| IBIS file stm32l4r5_s5_r7_s7_ufbga169.ibs
[IBIS ver]   4.2
[File name]   stm32l4r5_s5_r7_s7_ufbga169.ibs
[File Rev]   1.0
[Date]   01-6-2017
[Source]   Data Created at STMicroelectronics
[Notes]   File originated from ELDO simulations.
[Disclaimer]  This information is for modeling purpose only and is
   not guaranted.
   The information is subject to change without notice.
[Copyright]   Copyright 2017 STMicroelectronics Inc.
|   Component stm32l4r5_s5_r7_s7_ufbga169
[Component] stm32l4r5_s5_r7_s7_ufbga169
[Manufacturer] STMicroelectronics
[Package]
| variable   typ   min   max
R_pkg   0.0   0.0   0.0
L_pkg   0.0H   0.0H   0.0H
C_pkg   0.0F   0.0F   0.0F
[Pin]  signal_name   model_name   R_pin   L_pin   C_pin
A1 PI10 io8prog2m25m50m120m_sudq_ft
A10 PA14 io8prog2m25m50m120m_sudq_ft
A11 PA13 io8prog2m25m50m120m_sudq_ft
A12 PI0 io8prog2m25m50m120m_sudq_ft
A13 PH14 io8prog2m25m50m120m_sudq_ft
A2 PH2 io8prog2m25m50m120m_sudq_ft
A3 VDD power
A4 PE0 io8prog2m25m50m120m_sudq_ft
A5 PB4 io8prog2m25m50m120m_sudq_i2c_ft
A6 PB3 io8prog2m25m50m120m_sudq_ft
A7 VSS gnd
A8 VDD power
A9 PA15 io8prog2m25m50m120m_sudq_ft
B1 PI9 io8prog2m25m50m120m_sudq_ft
B10 PI2 io8prog2m25m50m120m_sudq_ft
B11 PI1 io8prog2m25m50m120m_sudq_ft
B12 PH15 io8prog2m25m50m120m_sudq_ft
B13 PH12 io8prog2m25m50m120m_sudq_ft
B2 PI7 io8prog2m25m50m120m_sudq_ft
B3 VSS gnd
B4 PE1 io8prog2m25m50m120m_sudq_ft
B5 PB5 io8prog2m25m50m120m_sudq_ft
B6 VDDIO2 power
B7 PG9 io8prog2m25m50m120m_sudq_ft
B8 PD0 io8prog2m25m50m120m_sudq_ft
B9 PI6 io8prog2m25m50m120m_sudq_ft
C1 VDD power
C10 PI3 io8prog2m25m50m120m_sudq_ft
C11 PI8 io8prog2m25m50m120m_sudq_ft
C12 VSS gnd
C13 VDD power
C2 VSS gnd
C3 PI11 io8prog2m25m50m120m_sudq_ft
C4 PB8 io8prog2m25m50m120m_sudq_i2c_ft
C5 PB6 io8prog2m25m50m120m_sudq_i2c_ft
C6 PG15 io8prog2m25m50m120m_sudq_ft
C7 PD4 io8prog2m25m50m120m_sudq_ft
C8 PD1 io8prog2m25m50m120m_sudq_ft
C9 PH13 io8prog2m25m50m120m_sudq_ft
D1 PE4 io8prog2m25m50m120m_sudq_ft
D10 PI4 io8prog2m25m50m120m_sudq_ft
D11 PH9 io8prog2m25m50m120m_sudq_ft
D12 PH7 io8prog2m25m50m120m_sudq_i2c_ft
D13 PA12 io8usblsfs_otg2
D2 PE3 io8prog2m25m50m120m_sudq_ft
D3 PE2 io8prog2m25m50m120m_sudq_ft
D4 PB9 io8prog2m25m50m120m_sudq_i2c_ft
D5 PB7 io8prog2m25m50m120m_sudq_i2c_ft
D6 PG10 io8prog2m25m50m120m_sudq_ft
D7 PD5 io8prog2m25m50m120m_sudq_ft
D8 PD2 io8prog2m25m50m120m_sudq_ft
D9 PC10 io8prog2m25m50m120m_sudq_ft
E1 PC13 io8prog2m25m50m120m_sudq_ft
E10 PI5 io8prog2m25m50m120m_sudq_ft
E11 PH6 io8prog2m25m50m120m_sudq_ft
E12 VDDUSB power
E13 PA11 io8usblsfs_otg2
E2 VBAT power
E3 PE6 io8prog2m25m50m120m_sudq_ft
E4 PE5 io8prog2m25m50m120m_sudq_ft
E5 PH3-BOOT0 io8prog2m25m50m120m_sudq_ft
E6 PG11 io8prog2m25m50m120m_sudq_ft
E7 PD6 io8prog2m25m50m120m_sudq_ft
E8 PD3 io8prog2m25m50m120m_sudq_ft
E9 PC11 io8prog2m25m50m120m_sudq_ft
F1 PC14-OSC32_IN io8prog2m25m50m120m_sudq_ft
F10 PA9 power
F11 PC6 io8prog2m25m50m120m_sudq_ft
F12 VDDIO2 power
F13 VSS gnd
F2 VSS gnd
F3 PF2 io8prog2m25m50m120m_sudq_ft
F4 PF1 io8prog2m25m50m120m_sudq_i2c_ft
F5 PF0 io8prog2m25m50m120m_sudq_i2c_ft
F6 PG12 io8prog2m25m50m120m_sudq_ft
F7 PD7 io8prog2m25m50m120m_sudq_ft
F8 PC12 io8prog2m25m50m120m_sudq_ft
F9 PA10 io8usb_id_otg20_lcd4_ft_ms
G1 PC15-OSC32_OUT io8prog2m25m50m120m_sudq_ft
G10 PC8 io8prog2m25m50m120m_sudq_ft
G11 PG6 io8prog2m25m50m120m_sudq_ft
G12 PC7 io8prog2m25m50m120m_sudq_ft
G13 VDD power
G2 VDD power
G3 PF3 io8prog2m25m50m120m_sudq_ft
G4 PF4 io8prog2m25m50m120m_sudq_ft
G5 PF5 io8prog2m25m50m120m_sudq_ft
G6 PG14 io8prog2m25m50m120m_sudq_i2c_ft
G7 PG13 io8prog2m25m50m120m_sudq_i2c_ft
G8 PA8 io8prog2m25m50m120m_sudq_ft
G9 PC9 io8prog2m25m50m120m_sudq_ft
H1 PH0-OSC_IN io8prog2m25m50m120m_sudq_ft
H10 PG7 io8prog2m25m50m120m_sudq_i2c_ft
H11 PD15 io8prog2m25m50m120m_sudq_ft
H12 VSS gnd
H13 VDD power
H2 VSS gnd
H3 NRST ioreset_ft_v33
H4 PF10 io8prog2m25m50m120m_sudq_ft
H5 PC4 io8prog2m25m50m120m_sudq_ft
H6 PG1 io8prog2m25m50m120m_sudq_ft
H7 PE10 io8prog2m25m50m120m_sudq_ft
H8 PB11 io8prog2m25m50m120m_sudq_i2c_ft
H9 PG8 io8prog2m25m50m120m_sudq_i2c_ft
J1 PH1-OSC_OUT io8prog2m25m50m120m_sudq_ft
J10 PG4 io8prog2m25m50m120m_sudq_ft
J11 PG3 io8prog2m25m50m120m_sudq_ft
J12 PG2 io8prog2m25m50m120m_sudq_ft
J13 PD10 io8prog2m25m50m120m_sudq_ft
J2 PC0 io8prog2m25m50m120m_sudq_i2c_ft
J3 PC1 io8prog2m25m50m120m_sudq_i2c_ft
J4 PC2 io8prog2m25m50m120m_sudq_ft
J5 PC5 io8prog2m25m50m120m_sudq_ft
J6 PG0 io8prog2m25m50m120m_sudq_ft
J7 PE9 io8prog2m25m50m120m_sudq_ft
J8 PE15 io8prog2m25m50m120m_sudq_ft
J9 PG5 io8prog2m25m50m120m_sudq_ft
K1 PC3 io8prog2m25m50m120m_sudq_ft
K10 PD14 io8prog2m25m50m120m_sudq_ft
K11 PD12 io8prog2m25m50m120m_sudq_ft
K12 PD11 io8prog2m25m50m120m_sudq_ft
K13 PD13 io8prog2m25m50m120m_sudq_ft
K2 VSSA/VREF- gnd
K3 PA0 io8prog2m25m50m120m_sudq_ft
K4 PA5 io8prog2m25m50m120m_sudq_ft
K5 PB0 io8prog2m25m50m120m_sudq_ft
K6 PF15 io8prog2m25m50m120m_sudq_i2c_ft
K7 PE8 io8prog2m25m50m120m_sudq_ft
K8 PE14 io8prog2m25m50m120m_sudq_ft
K9 PH4 io8prog2m25m50m120m_sudq_i2c_ft
L1 VREF+ power
L10 PD9 io8prog2m25m50m120m_sudq_ft
L11 PD8 io8prog2m25m50m120m_sudq_ft
L12 VDD power
L13 VSS gnd
L2 VDDA power
L3 PA4 io8prog2m25m50m120m_sudq_ft
L4 PA7 io8prog2m25m50m120m_sudq_i2c_ft
L5 PB1 io8prog2m25m50m120m_sudq_ft
L6 PF14 io8prog2m25m50m120m_sudq_i2c_ft
L7 PE7 io8prog2m25m50m120m_sudq_ft
L8 PE13 io8prog2m25m50m120m_sudq_ft
L9 PH5 io8prog2m25m50m120m_sudq_i2c_ft
M1 OPAMP1_VINM NC
M10 PH11 io8prog2m25m50m120m_sudq_ft
M11 VSS gnd
M12 PB15 io8prog2m25m50m120m_sudq_ft
M13 PB14 io8prog2m25m50m120m_sudq_i2c_ft
M2 PA3 io8prog2m25m50m120m_sudq_ft
M3 VSS gnd
M4 PA6 io8prog2m25m50m120m_sudq_ft
M5 PF11 io8prog2m25m50m120m_sudq_ft
M6 PF13 io8prog2m25m50m120m_sudq_ft
M7 VSS gnd
M8 PE12 io8prog2m25m50m120m_sudq_ft
M9 PH10 io8prog2m25m50m120m_sudq_ft
N1 PA2 io8prog2m25m50m120m_sudq_ft
N10 PH8 io8prog2m25m50m120m_sudq_i2c_ft
N11 VDD power
N12 PB12 io8prog2m25m50m120m_sudq_ft
N13 PB13 io8prog2m25m50m120m_sudq_i2c_ft
N2 PA1 io8prog2m25m50m120m_sudq_ft
N3 VDD power
N4 OPAMP2_VINM NC
N5 PB2 io8prog2m25m50m120m_sudq_ft
N6 PF12 io8prog2m25m50m120m_sudq_ft
N7 VDD power
N8 PE11 io8prog2m25m50m120m_sudq_ft
N9 PB10 io8prog2m25m50m120m_sudq_i2c_ft
[Diff Pin]   inv_pin   vdiff   tdelay_typ  tdelay_min  tdelay_max
D13 E13 200mV   NA   NA   NA
[Model Selector] io8prog2m25m50m120m_sudq_ft
io8p00_sudq_ft_pd_lv  "SPEED00, PD=40kOhm - 1P8V"
io8p00_sudq_ft_pu_lv  "SPEED00, PU=40kOhm - 1P8V"
io8p00_sudq_ft_lv  "SPEED00 - 1P8V"
io8p00_sudq_ft_pd  "SPEED00, PD=40kOhm - 3P3V"
io8p00_sudq_ft_pu  "SPEED00, PU=40kOhm - 3P3V"
io8p00_sudq_ft  "SPEED00 - 3P3V"
io8p01_sudq_ft_pd_lv  "SPEED01, PD=40kOhm - 1P8V"
io8p01_sudq_ft_pu_lv  "SPEED01, PU=40kOhm - 1P8V"
io8p01_sudq_ft_lv  "SPEED01 - 1P8V"
io8p01_sudq_ft_pd  "SPEED01, PD=40kOhm - 3P3V"
io8p01_sudq_ft_pu  "SPEED01, PU=40kOhm - 3P3V"
io8p01_sudq_ft  "SPEED01 - 3P3V"
io8p10_sudq_ft_pd_lv  "SPEED10, PD=40kOhm - 1P8V"
io8p10_sudq_ft_pu_lv  "SPEED10, PU=40kOhm - 1P8V"
io8p10_sudq_ft_lv  "SPEED10 - 1P8V"
io8p10_sudq_ft_pd  "SPEED10, PD=40kOhm - 3P3V"
io8p10_sudq_ft_pu  "SPEED10, PU=40kOhm - 3P3V"
io8p10_sudq_ft  "SPEED10 - 3P3V"
io8p11_sudq_ft_pd_lv  "SPEED11, PD=40kOhm - 1P8V"
io8p11_sudq_ft_pu_lv  "SPEED11, PU=40kOhm - 1P8V"
io8p11_sudq_ft_lv  "SPEED11 - 1P8V"
io8p11_sudq_ft_pd  "SPEED11, PD=40kOhm - 3P3V"
io8p11_sudq_ft_pu  "SPEED11, PU=40kOhm - 3P3V"
io8p11_sudq_ft  "SPEED11 - 3P3V"
[Model Selector] io8prog2m25m50m120m_sudq_i2c_ft
io8prog_1v8_i2c_pd  "5V Tol GPIO 1.8V range i2c functionality with pull down"
io8prog_1v8_i2c_pu  "5V Tol GPIO 1.8V range i2c functionality with pull up"
io8prog_1v8_i2c  "5V Tol GPIO 1.8V range i2c functionality"
io8prog_3v3_i2c_pd  "5V Tol GPIO 3.3V range i2c functionality with pull down"
io8prog_3v3_i2c_pu  "5V Tol GPIO 3.3V range i2c functionality with pull up"
io8prog_3v3_i2c  "5V Tol GPIO 3.3V range i2c functionality"
io8prog_1v8_pd_00  "5V Tol GPIO 1.8V range with pd speed 00"
io8prog_1v8_pu_00  "5V Tol GPIO 1.8V range with pu speed 00"
io8prog_1v8_00  "5V Tol GPIO 1.8V range speed 00"
io8prog_3v3_pd_00  "5V Tol GPIO 3.3V range with pd speed 00"
io8prog_3v3_pu_00  "5V Tol GPIO 3.3V range with pu speed 00"
io8prog_3v3_00  "5V Tol GPIO 3.3V range speed 00"
io8prog_1v8_pd_01  "5V Tol GPIO 1.8V range with pd speed 01"
io8prog_1v8_pu_01  "5V Tol GPIO 1.8V range with pu speed 01"
io8prog_1v8_01  "5V Tol GPIO 1.8V range speed 01"
io8prog_3v3_pd_01  "5V Tol GPIO 3.3V range with pd speed 01"
io8prog_3v3_pu_01  "5V Tol GPIO 3.3V range with pu speed 01"
io8prog_3v3_01  "5V Tol GPIO 3.3V range speed 01"
io8prog_1v8_pd_10  "5V Tol GPIO 1.8V range with pd speed 10"
io8prog_1v8_pu_10  "5V Tol GPIO 1.8V range with pu speed 10"
io8prog_1v8_10  "5V Tol GPIO 1.8V range speed 10"
io8prog_3v3_pd_10  "5V Tol GPIO 3.3V range with pd speed 10"
io8prog_3v3_pu_10  "5V Tol GPIO 3.3V range with pu speed 10"
io8prog_3v3_10  "5V Tol GPIO 3.3V range speed 10"
io8prog_1v8_pd_11  "5V Tol GPIO 1.8V range with pd speed 11"
io8prog_1v8_pu_11  "5V Tol GPIO 1.8V range with pu speed 11"
io8prog_1v8_11  "5V Tol GPIO 1.8V range speed 11"
io8prog_3v3_pd_11  "5V Tol GPIO 3.3V range with pd speed 11"
io8prog_3v3_pu_11  "5V Tol GPIO 3.3V range with pu speed 11"
io8prog_3v3_11  "5V Tol GPIO 3.3V range speed 11"
[Model Selector] io8usb_id_otg20_lcd4_ft_ms
io8usbid_1v8_id_pu  "ID 1V8 range with pull up"
io8usbid_3v3_id_pu  "ID 3V3 range with pull up"
io8usbid_1v8_id  "ID 1V8 range"
io8usbid_3v3_id  "ID 3V3 range"
io8usbid_1v8_pd_00  "GPIO 1.8V range with pd speed 00"
io8usbid_1v8_pu_00  "GPIO 1.8V range with pu speed 00"
io8usbid_1v8_00  "GPIO 1.8V range speed 00"
io8usbid_3v3_pd_00  "GPIO 3.3V range with pd speed 00"
io8usbid_3v3_pu_00  "GPIO 3.3V range with pu speed 00"
io8usbid_3v3_00  "GPIO 3.3V range speed 00"
io8usbid_1v8_pd_01  "GPIO 1.8V range with pd speed 01"
io8usbid_1v8_pu_01  "GPIO 1.8V range with pu speed 01"
io8usbid_1v8_01  "GPIO 1.8V range speed 01"
io8usbid_3v3_pd_01  "GPIO 3.3V range with pd speed 01"
io8usbid_3v3_pu_01  "GPIO 3.3V range with pu speed 01"
io8usbid_3v3_01  "GPIO 3.3V range speed 01"
io8usbid_1v8_pd_10  "GPIO 1.8V range with pd speed 10"
io8usbid_1v8_pu_10  "GPIO 1.8V range with pu speed 10"
io8usbid_1v8_10  "GPIO 1.8V range speed 10"
io8usbid_3v3_pd_10  "GPIO 3.3V range with pd speed 10"
io8usbid_3v3_pu_10  "GPIO 3.3V range with pu speed 10"
io8usbid_3v3_10  "GPIO 3.3V range speed 10"
io8usbid_1v8_pd_11  "GPIO 1.8V range with pd speed 11"
io8usbid_1v8_pu_11  "GPIO 1.8V range with pu speed 11"
io8usbid_1v8_11  "GPIO 1.8V range speed 11"
io8usbid_3v3_pd_11  "GPIO 3.3V range with pd speed 11"
io8usbid_3v3_pu_11  "GPIO 3.3V range with pu speed 11"
io8usbid_3v3_11  "GPIO 3.3V range speed 11"
[Model Selector] io8usblsfs_otg2
usb_ls_pd  "USB Low Speed mode - Pull Down"
usb_ls_pu2  "USB Low Speed mode - Pull up 2"
usb_ls_pu  "USB Low Speed mode - Pull up"
usb_fs  "USB Low Speed mode"
usb_fs_pd  "USB Full Speed mode - Pull Down"
usb_fs_pu2  "USB Full Speed mode - Pull up 2"
usb_fs_pu  "USB Full Speed mode - Pull up"
[Model Selector] ioreset_ft_v33
ioreset_1v2_pu  "RESET 1.2V range with PU"
ioreset_1v2  "RESET 1.2V range"
ioreset_1v8_pu  "RESET 1.8V range with PU"
ioreset_1v8  "RESET 1.8V range"
ioreset_3v3_pu  "RESET 3.3V range with PU"
ioreset_3v3  "RESET 3.3V range"
| Models and submodels in the file (95): io8p00_sudq_ft_pd_lv (I/O), io8p00_sudq_ft_pu_lv (I/O), io8p00_sudq_ft_lv (I/O), io8p00_sudq_ft_pd (I/O), io8p00_sudq_ft_pu (I/O), io8p00_sudq_ft (I/O), io8p01_sudq_ft_pd_lv (I/O), io8p01_sudq_ft_pu_lv (I/O), io8p01_sudq_ft_lv (I/O), io8p01_sudq_ft_pd (I/O), io8p01_sudq_ft_pu (I/O), io8p01_sudq_ft (I/O), io8p10_sudq_ft_pd_lv (I/O), io8p10_sudq_ft_pu_lv (I/O), io8p10_sudq_ft_lv (I/O), io8p10_sudq_ft_pd (I/O), io8p10_sudq_ft_pu (I/O), io8p10_sudq_ft (I/O), io8p11_sudq_ft_pd_lv (I/O), io8p11_sudq_ft_pu_lv (I/O), io8p11_sudq_ft_lv (I/O), io8p11_sudq_ft_pd (I/O), io8p11_sudq_ft_pu (I/O), io8p11_sudq_ft (I/O), io8prog_1v8_i2c_pd (I/O), io8prog_1v8_i2c_pu (I/O), io8prog_1v8_i2c (I/O), io8prog_3v3_i2c_pd (I/O), io8prog_3v3_i2c_pu (I/O), io8prog_3v3_i2c (I/O), io8prog_1v8_pd_00 (I/O), io8prog_1v8_pu_00 (I/O), io8prog_1v8_00 (I/O), io8prog_3v3_pd_00 (I/O), io8prog_3v3_pu_00 (I/O), io8prog_3v3_00 (I/O), io8prog_1v8_pd_01 (I/O), io8prog_1v8_pu_01 (I/O), io8prog_1v8_01 (I/O), io8prog_3v3_pd_01 (I/O), io8prog_3v3_pu_01 (I/O), io8prog_3v3_01 (I/O), io8prog_1v8_pd_10 (I/O), io8prog_1v8_pu_10 (I/O), io8prog_1v8_10 (I/O), io8prog_3v3_pd_10 (I/O), io8prog_3v3_pu_10 (I/O), io8prog_3v3_10 (I/O), io8prog_1v8_pd_11 (I/O), io8prog_1v8_pu_11 (I/O), io8prog_1v8_11 (I/O), io8prog_3v3_pd_11 (I/O), io8prog_3v3_pu_11 (I/O), io8prog_3v3_11 (I/O), io8usbid_1v8_id_pu (Input), io8usbid_3v3_id_pu (Input), io8usbid_1v8_id (Input), io8usbid_3v3_id (Input), io8usbid_1v8_pd_00 (I/O), io8usbid_1v8_pu_00 (I/O), io8usbid_1v8_00 (I/O), io8usbid_3v3_pd_00 (I/O), io8usbid_3v3_pu_00 (I/O), io8usbid_3v3_00 (I/O), io8usbid_1v8_pd_01 (I/O), io8usbid_1v8_pu_01 (I/O), io8usbid_1v8_01 (I/O), io8usbid_3v3_pd_01 (I/O), io8usbid_3v3_pu_01 (I/O), io8usbid_3v3_01 (I/O), io8usbid_1v8_pd_10 (I/O), io8usbid_1v8_pu_10 (I/O), io8usbid_1v8_10 (I/O), io8usbid_3v3_pd_10 (I/O), io8usbid_3v3_pu_10 (I/O), io8usbid_3v3_10 (I/O), io8usbid_1v8_pd_11 (I/O), io8usbid_1v8_pu_11 (I/O), io8usbid_1v8_11 (I/O), io8usbid_3v3_pd_11 (I/O)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
